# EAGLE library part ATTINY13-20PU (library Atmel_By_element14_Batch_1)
8-bit MCU
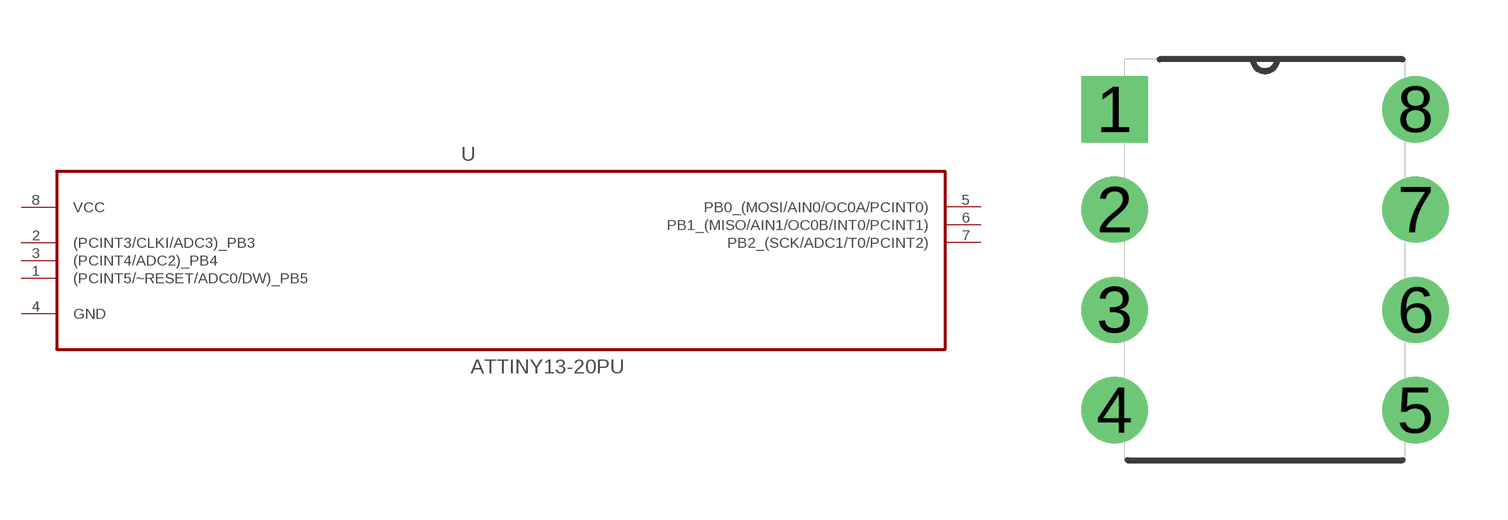
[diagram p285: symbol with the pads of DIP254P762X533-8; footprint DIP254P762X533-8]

Designator prefix U

## ATTINY13-20PU (MPN: ATTINY13-20PU; OC_FARNELL: 9171550; OC_NEWARK: 96K6521; PACKAGE: DIP-8; SUPPLIER: Atmel)  [DIP254P762X533-8]
1  (PCINT5/~RESET/ADC0/DW)_PB5
2  (PCINT3/CLKI/ADC3)_PB3
3  (PCINT4/ADC2)_PB4
4  GND  pas
5  PB0_(MOSI/AIN0/OC0A/PCINT0)
6  PB1_(MISO/AIN1/OC0B/INT0/PCINT1)
7  PB2_(SCK/ADC1/T0/PCINT2)
8  VCC  pwr

## Footprint DIP254P762X533-8 (pad centres in mm)
drill 1.118 square: 1 -7.62,7.62
drill 1.118: 2 -7.62,5.08; 3 -7.62,2.54; 4 -7.62,0; 5 0,0; 6 0,2.54; 7 0,5.08; 8 0,7.62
